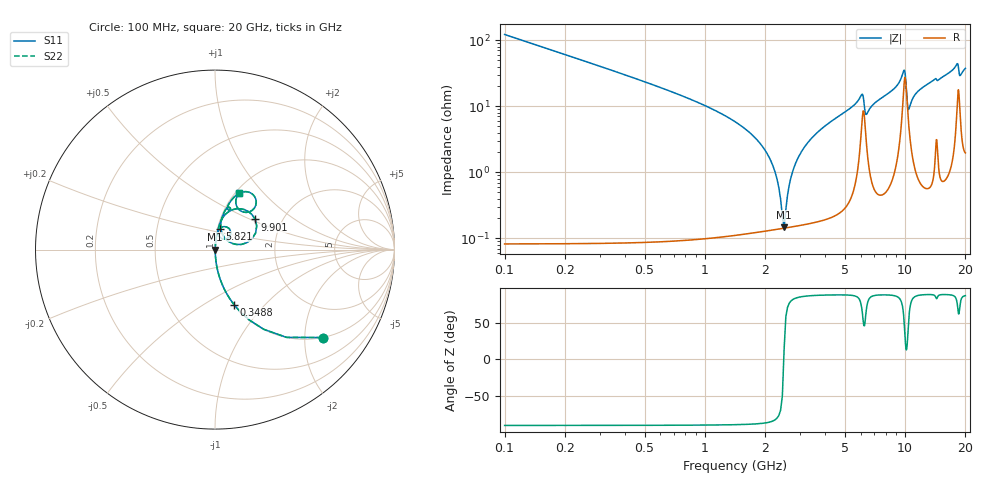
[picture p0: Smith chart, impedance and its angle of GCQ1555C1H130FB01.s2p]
!Murata Part Number: GCQ1555C1H130FB01
!These Parameters are Measured in Series Mode Connection
!Data Generated on Mar 13, 2026
!  o--ll--o
!Port1  Port2
!  o------o
!Operation Temp=25[degC], DC Bias Voltage=0[V]
!Freq. Start=100[MHz] Stop=20[GHz] 401[Steps]
# Hz S RI R 50
!Freq.(Hz) S11(Real) S11(Imag) S21(Real) S21(Imag) S12(Real) S12(Imag) S22(Real) S22(Imag)
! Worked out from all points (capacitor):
!   401 points, 100 MHz to 20 GHz, reference 50 ohm
!   read as one part in series: C = 13 pF near 199.5 MHz
!   lowest |Z| = 147 mohm at 2.488 GHz (marker M1)
!   series resonance near 2.479 GHz, so ESL is about 320 pH
!   S11 on the Smith chart (normalised r, x): 100 MHz: 1.00, -2.44; 348.8 MHz: 1.00, -0.69; 5.821 GHz: 1.02, +0.24; 9.901 GHz: 1.46, +0.53; 20 GHz: 1.04, +0.75
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1e8  0.599 -0.4898  0.401 0.4898  0.401 0.4898  0.599 -0.4898
3.4875e8  0.1065 -0.3072  0.8935 0.3072  0.8935 0.3072  0.1065 -0.3072
1.94075e9  0.00186 -0.0244  0.9981 0.0244  0.9981 0.0244  0.00186 -0.0244
2.1895e9  0.00149 -0.0123  0.9985 0.0123  0.9985 0.0123  0.00149 -0.0123
2.3885e9  0.00141 -0.00369  0.9986 0.00369  0.9986 0.00369  0.00141 -0.00369
2.488e9  0.00142 0.000362  0.9986 -0.000362  0.9986 -0.000362  0.00142 0.000362
2.83625e9  0.0017 0.0134  0.9983 -0.0134  0.9983 -0.0134  0.0017 0.0134
3.43325e9  0.00281 0.0333  0.9972 -0.0333  0.9972 -0.0333  0.00281 0.0333
5.82125e9  0.0259 0.1164  0.9741 -0.1164  0.9741 -0.1164  0.0259 0.1164
6.11975e9  0.0797 0.1167  0.9203 -0.1167  0.9203 -0.1167  0.0797 0.1167
6.41825e9  0.03 0.0671  0.97 -0.0671  0.97 -0.0671  0.03 0.0671
6.7665e9  0.017 0.0957  0.983 -0.0957  0.983 -0.0957  0.017 0.0957
9.1545e9  0.0562 0.1945  0.9438 -0.1945  0.9438 -0.1945  0.0562 0.1945
9.90075e9  0.2242 0.1678  0.7758 -0.1678  0.7758 -0.1678  0.2242 0.1678
1.005e10  0.2055 0.0593  0.7945 -0.0593  0.7945 -0.0593  0.2055 0.0593
1.039825e10  0.0581 0.061  0.9419 -0.061  0.9419 -0.061  0.0581 0.061
1.13435e10  0.0329 0.15  0.9671 -0.15  0.9671 -0.15  0.0329 0.15
1.338325e10  0.0553 0.2159  0.9447 -0.2159  0.9447 -0.2159  0.0553 0.2159
1.67165e10  0.1043 0.2901  0.8957 -0.2901  0.8957 -0.2901  0.1043 0.2901
1.835825e10  0.2299 0.2646  0.7701 -0.2646  0.7701 -0.2646  0.2299 0.2646
1.875625e10  0.1385 0.219  0.8615 -0.219  0.8615 -0.219  0.1385 0.219
2e10  0.1359 0.3174  0.8641 -0.3174  0.8641 -0.3174  0.1359 0.3174
